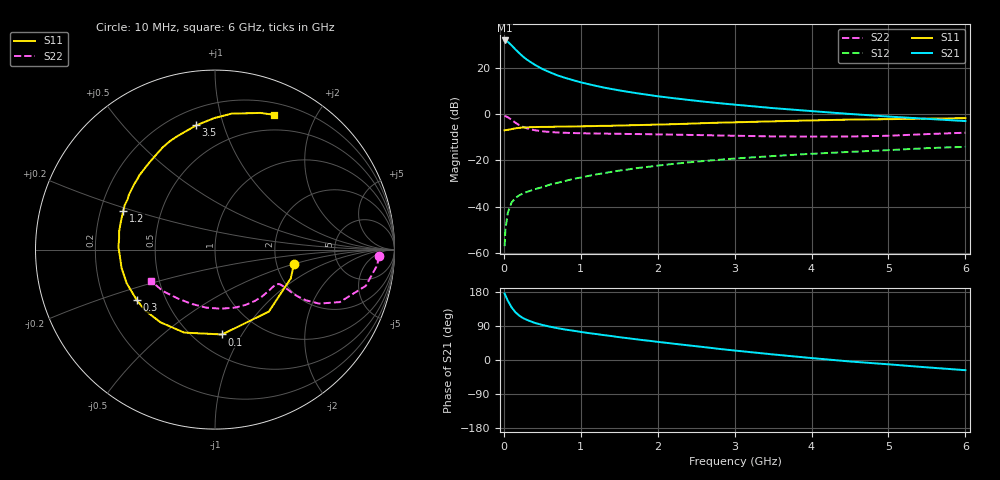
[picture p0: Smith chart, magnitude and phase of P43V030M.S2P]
! SIEMENS Small Signal Semiconductors
! BFP182
! Si NPN RF Bipolar Junction Transistor in SOT143
! VCE = 3 V  IC = 30 mA
! Common Emitter S-Parameters:  March  1996
# GHz  S  MA  R  50
!  f  S11  S21  S12  S22
! GHz  MAG  ANG  MAG  ANG  MAG  ANG  MAG  ANG
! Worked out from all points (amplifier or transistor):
!   36 points, 10 MHz to 6 GHz, reference 50 ohm
!   highest |S21| = 31.9 dB at 10 MHz (marker M1)
!   |S21| within 3 dB of that: start of sweep to 125.7 MHz
!   unconditionally stable (mu >= 1): start of sweep to 11.9 MHz; 438.9 MHz to 5.953 GHz
!   at 250 MHz: K = 0.72, MSG = 29.6 dB, |S12| = -34.3 dB
!   at 1.4 GHz: K = 1.37, MAG = 14.3 dB, |S12| = -24.9 dB
!   at 6 GHz: K = 1.00, MSG = 5.6 dB, |S12| = -14.1 dB
!   S11 on the Smith chart (normalised r, x): 10 MHz: 2.50, -0.50; 100 MHz: 0.68, -0.83; 300 MHz: 0.34, -0.26; 1.2 GHz: 0.30, +0.19; 3.5 GHz: 0.30, +0.81; 6 GHz: 0.32, +1.48
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0.01  0.4473 -10.2  39.26 175.2  0.0014 84.8  0.9131 -2.4
0.02  0.4517 -20.8  39.25 170.7  0.0031 83.6  0.908 -5.5
0.05  0.4574 -49.0  37 157.1  0.0072 79.0  0.8641 -13.5
0.1  0.4745 -85.2  30.8 139.1  0.0123 60.5  0.7544 -22.8
0.15  0.4933 -110.4  25.23 126.2  0.0154 54.5  0.6537 -27.4
0.2  0.5062 -126.8  20.93 117.2  0.0176 52.5  0.5815 -29.1
0.25  0.5158 -138.4  17.56 110.6  0.0193 49.7  0.5303 -29.5
0.3  0.5189 -147.0  15.11 105.8  0.0208 50.0  0.494 -29.3
0.4  0.5266 -159.3  11.76 98.0  0.0238 51.8  0.4504 -28.5
0.5  0.5306 -169.0  9.512 92.5  0.0264 52.4  0.4262 -28.2
0.6  0.5311 -175.8  8.024 87.9  0.03 55.4  0.4119 -28.1
0.7  0.5382 178.5  6.871 83.9  0.0329 56.0  0.402 -28.5
0.8  0.538 173.3  6.078 80.3  0.0361 56.8  0.3957 -29.2
1.1  0.5496 160.7  4.462 71.1  0.0463 58.2  0.3842 -32.5
1.2  0.5545 157.0  4.084 68.5  0.0498 58.0  0.3821 -33.9
1.7  0.5796 140.8  2.887 55.2  0.0672 56.3  0.3719 -42.2
2.2  0.6075 127.0  2.223 43.2  0.084 53.0  0.3621 -52.2
2.8  0.6545 112.5  1.727 29.3  0.1034 47.6  0.3457 -65.8
3.5  0.7003 98.6  1.352 14.7  0.1243 41.3  0.3308 -84.4
4.5  0.7633 83.0  1.011 -3.9  0.1532 32.5  0.3294 -113.4
5.5  0.8021 71.7  0.793 -19.4  0.1844 23.8  0.3707 -141.3
6  0.8201 66.3  0.71 -26.9  0.1967 18.4  0.3977 -154.0
